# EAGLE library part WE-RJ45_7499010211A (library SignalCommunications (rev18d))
Order Code 7499010211A Design THT xBase-T 10/100 Base-T Ports 1x1 Application Standard Tab Position DOWN LED (Left-Right) Green-Yellow EMI Fingers No Details see: http://katalog.we-online.de/en/pbs/WE-LAN_RJ45/7499010211A? Updated by Yingchun Shan 2016-08-26 2016(C) Würth Elektronik
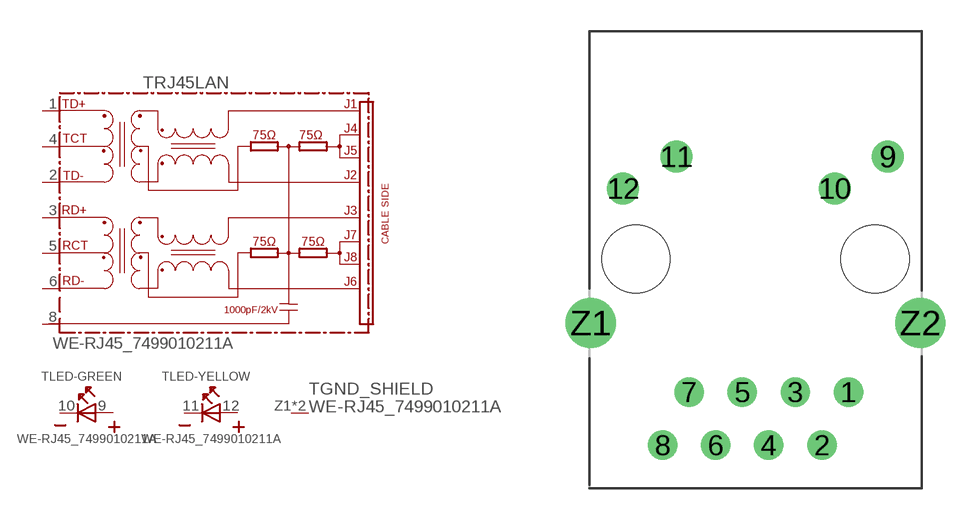
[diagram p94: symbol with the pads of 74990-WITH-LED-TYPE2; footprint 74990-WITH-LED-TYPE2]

Designator prefix T; gates RJ45LAN=74990X-THT-10/100-T LED-GREEN=LED2PIN LED-YELLOW=LED2PIN GND_SHIELD=GND_PIN

## WE-RJ45_7499010211A (COMPANY-URL: http://www.we-online.de; CREATED-BY: Christin Zierenner; CREATED-DATE: AUG 2012; DATASHEET-URL: http://katalog.we-online.de/kataloge/eisos/media/pdf/7499010211A.pdf; MANUFACTURER: Würth Elektronik eiSos GmbH)  [74990-WITH-LED-TYPE2]
1  RJ45LAN:TD+
2  RJ45LAN:TD-
3  RJ45LAN:RD+
4  RJ45LAN:TCT
5  RJ45LAN:RCT
6  RJ45LAN:RD-
8  RJ45LAN:8
9  LED-GREEN:A  pas
10  LED-GREEN:K  pas
11  LED-YELLOW:K  pas
12  LED-YELLOW:A  pas
Z1  GND_SHIELD:1  pwr
Z2  GND_SHIELD:1  pwr

## Footprint 74990-WITH-LED-TYPE2 (pad centres in mm)
MAX HEIGHT=13.50mm PORTS----1X1 LED ----YES
drill 0.9: 1 4.445,-6.35; 2 3.175,-8.89; 3 1.905,-6.35; 4 0.635,-8.89; 5 -0.635,-6.35; 6 -1.905,-8.89; 7 -3.175,-6.35; 8 -4.445,-8.89
drill 1.02: 9 6.325,4.9; 10 3.785,3.38; 11 -3.785,4.9; 12 -6.325,3.38
drill 1.6: Z1 -7.875,-3.05; Z2 7.875,-3.05
hole 3.25 at 5.715,0
hole 3.25 at -5.715,0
